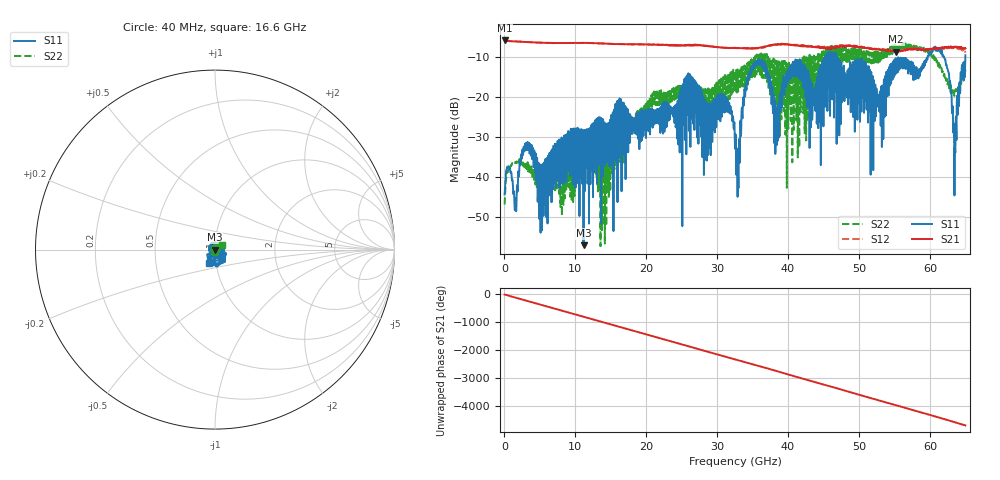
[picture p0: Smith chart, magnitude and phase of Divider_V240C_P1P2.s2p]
! Created Tue Jul 15 20:13:44 2008
# hz S ma R 50
! 2 Port Network Data from blockName block
! freq  magS11  angS11  magS21  angS21  magS12  angS12  magS22  angS22
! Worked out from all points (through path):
!   1601 points, 40 MHz to 65 GHz, reference 50 ohm
!   highest |S21| = -6.01 dB at 40 MHz (marker M1); lowest = -8.8 dB at 55.22 GHz (marker M2)
!   group delay of S21, straight-line fit = 200 ps
!   lowest |S11| = -56.9 dB at 11.16 GHz (marker M3), VSWR 1.00, Z = 49.9 + j0.0358 ohm
!   |S11| at or under -10 dB: start of sweep to 45.26 GHz; 46.78 GHz to 59.7 GHz (12.91 GHz wide, 24.3 % of centre); 61.96 GHz to 64.99 GHz (3.035 GHz wide, 4.78 % of centre)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
!   |S22| runs from -57.2 to -6.7 dB; largest |S21 - S12| = 0.053
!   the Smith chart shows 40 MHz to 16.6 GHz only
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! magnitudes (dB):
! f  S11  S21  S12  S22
! 40 MHz  -44.3  -6.0  -6.0  -46.8
! 1.583 GHz  -45.2  -6.2  -6.2  -36.2
! 3.207 GHz  -33.2  -6.4  -6.4  -38.0
! 5.196 GHz  -37.1  -6.6  -6.6  -43.1
! 10.88 GHz  -28.1  -6.6  -6.6  -38.1
! 11.16 GHz  -56.9  -6.6  -6.6  -30.4
! 13.88 GHz  -28.0  -6.7  -6.7  -35.7
! 21.72 GHz  -23.0  -7.1  -7.1  -18.5
! 26.23 GHz  -32.5  -7.1  -7.1  -16.1
! 32.52 GHz  -32.9  -7.9  -7.8  -15.3
! 33.01 GHz  -42.7  -7.9  -7.9  -15.4
! 33.94 GHz  -20.0  -7.9  -7.9  -17.7
! 35.65 GHz  -12.1  -7.9  -7.9  -10.2
! 38.33 GHz  -22.8  -7.0  -7.1  -12.1
! 40.76 GHz  -14.3  -7.1  -7.2  -17.6
! 43.36 GHz  -19.3  -7.5  -7.4  -17.3
! 45.92 GHz  -24.8  -7.7  -7.7  -11.2
! 54.2 GHz  -15.1  -8.6  -8.4  -7.9
! 55.22 GHz  -11.4  -8.8  -8.5  -7.2
! 61.43 GHz  -8.4  -7.8  -8.0  -12.1
! 63.42 GHz  -31.9  -7.6  -7.8  -19.6
! 65 GHz  -9.7  -8.0  -9.0  -13.2
